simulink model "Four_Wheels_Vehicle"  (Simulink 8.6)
settings: Solver=ode45  StartTime=0.0  StopTime=20  RelTol=1e-3
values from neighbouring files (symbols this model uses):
  beta = 1    [Vehicle_Parameters.m]
  g = 9.81    [Vehicle_Parameters.m]
  H_CoG = 0.700    (= 0.7)    [Vehicle_Parameters.m]
  Hearo = 0.750    (= 0.75)    [Vehicle_Parameters.m]
  Iz = 2480    [Vehicle_Parameters.m]
  Jw = 2.166    [Vehicle_Parameters.m]
  L = 10    [Vehicle_Parameters.m]
  Lf = 1.180    (= 1.18)    [Vehicle_Parameters.m]
  Lr = 1.770    (= 1.77)    [Vehicle_Parameters.m]
  Lw = 1.880    (= 1.88)    [Vehicle_Parameters.m]
  m = 1500    [Vehicle_Parameters.m]
  miu = 0.85    [Vehicle_Parameters.m]
  reff = 0.380    (= 0.38)    [Vehicle_Parameters.m]
undefined symbols (not defined in the file or in its folder): DiscIntNeverNeededParam, Init, Ki, Kp, LowerLimit, sigbuilder_block, Ts, UpperLimit
libraries: simulink x15, powerlib_extras x3
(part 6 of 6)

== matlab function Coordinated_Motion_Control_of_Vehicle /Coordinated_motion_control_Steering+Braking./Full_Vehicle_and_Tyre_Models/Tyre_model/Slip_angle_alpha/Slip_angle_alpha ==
% =================================================================================================================================
% Function: Slip_angle_alpha
% Version:  0.00
% Since:    25 May 2016
% Author:   T.C. Lin
% Input:	x_Vel, y_Vel, yaw_rate, Lf, Lr, deltaw
% Output:	alpha_FL, alpha_FR, alpha_RL, alpha_RR
% Timing:   TBD
% Description: NA
% =================================================================================================================================

function [alpha_FL, alpha_FR, alpha_RL, alpha_RR] = Slip_angle(x_Vel, y_Vel, yaw_rate, Lf, Lr, deltaw)
%# codegen

% % ===== Slip angles at the front tire =====
% 
% % Slip angles at the front left tire
% alpha_FL = deltaw-atan(y_Vel+Lf*yaw_rate/x_Vel);
% 
% % Slip angles at the front right tire
% alpha_FR = deltaw-atan(y_Vel+Lf*yaw_rate/x_Vel);
% 
% 
% % ===== Slip angles at the rear tire =====
% 
% % Slip angles at the rear left tire
% alpha_RL = -atan(y_Vel-Lr*yaw_rate/x_Vel);
% 
% % Slip angles at the rear right tire
% alpha_RR = -atan(y_Vel-Lr*yaw_rate/x_Vel);



alpha_FL=deltaw-atan((y_Vel+Lf*yaw_rate)/(x_Vel-1.65*yaw_rate/2));
alpha_FR=deltaw-atan((y_Vel+Lf*yaw_rate)/(x_Vel+1.65*yaw_rate/2));
alpha_RL=-atan((y_Vel-Lr*yaw_rate)/(x_Vel-1.65*yaw_rate/2));
alpha_RR=-atan((y_Vel-Lr*yaw_rate)/(x_Vel+1.65*yaw_rate/2));

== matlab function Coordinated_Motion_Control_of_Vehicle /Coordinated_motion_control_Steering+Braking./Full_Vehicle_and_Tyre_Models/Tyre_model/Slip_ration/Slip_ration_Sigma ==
% =================================================================================================================================
% Function: Slip_Ration_Sigma
% Version:  0.00
% Since:    24 May 2016
% Author:   T.C. Lin
% Input:	Omega_FL, Omega_FR, Omega_RL, Omega_RR, x_Vel, reff
% Output:	Sigma_FL, Sigma_FR, Sigma_RL, Sigma_RR
% Timing:   TBD
% Description: NA
% =================================================================================================================================

function [Sigma_FL, Sigma_FR, Sigma_RL, Sigma_RR] = Slip_Ration(Omega_FL, Omega_FR, Omega_RL, Omega_RR, x_Vel, reff)
%#codegen

Sigma_FL = (reff*Omega_FL - x_Vel)/(x_Vel);
Sigma_FR = (reff*Omega_FR - x_Vel)/(x_Vel);

Sigma_RL = (reff*Omega_RL - x_Vel)/(x_Vel);
Sigma_RR = (reff*Omega_RR - x_Vel)/(x_Vel);

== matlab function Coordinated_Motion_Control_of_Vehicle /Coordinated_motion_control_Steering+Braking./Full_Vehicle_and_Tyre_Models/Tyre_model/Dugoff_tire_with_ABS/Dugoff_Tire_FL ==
% ================================================================================
% Function: Dugoff_Tire_FL
% Version:  0.00
% Since:    24 May 2016
% Author:   T.C. Lin
% Input:	Sigma, Fz_FL, alpha_FL, miu
% Output:	Fx_FL, Fy_FL
% Timing:   TBD
% Description: NA
% ================================================================================

function [Fx_FL, Fy_FL] = Dugoff_Tire_FL(Sigma, Fz_FL, alpha_FL, miu)
%# codegen

% Cornering stiffness of the tire
Cs = 20000;

% Longitudinal stiffness of the tire
C_alpha = 80000;

% Dugoff's tire model with a variable lamda in the wheel model
Lamda = miu*Fz_FL*(1+Sigma)/(2*sqrt((Cs*Sigma)^2+(C_alpha*(tan(alpha_FL)))^2));

if Lamda < 1
    
    f = Lamda*(2-Lamda);
    
else
    f = 1;
    
end

% Longitudinal tire force
Fx_FL = Cs*Sigma*f/(1+Sigma);

% Lateral tire force
Fy_FL = C_alpha*tan(alpha_FL)*f/(1+Sigma);

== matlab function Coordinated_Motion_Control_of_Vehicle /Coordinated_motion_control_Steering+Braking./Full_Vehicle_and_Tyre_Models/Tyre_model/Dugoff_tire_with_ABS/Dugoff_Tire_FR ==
% ================================================================================
% Function: Dugoff_Tire_FR
% Version:  0.00
% Since:    24 May 2016
% Author:   T.C. Lin
% Input:	Sigma, Fz_FL, alpha_FL, miu
% Output:	Fx_FL, Fy_FL
% Timing:   TBD
% Description: NA
% ================================================================================

function [Fx_FR, Fy_FR] = Dugoff_Tire_FR(Sigma, Fz_FR, alpha_FR, miu)
%# codegen

% Cornering stiffness of the tire
Cs = 20000;

% Longitudinal stiffness of the tire
C_alpha = 80000;

% Dugoff's tire model with a variable lamda in the wheel model
Lamda = miu*Fz_FR*(1+Sigma)/(2*sqrt((Cs*Sigma)^2+(C_alpha*(tan(alpha_FR)))^2));

if Lamda < 1
    
    f = Lamda*(2-Lamda);
    
else   
    f = 1;
    
end

% Longitudinal tire force
Fx_FR = Cs*Sigma*f/(1+Sigma);

% Lateral tire force
Fy_FR = C_alpha*tan(alpha_FR)*f/(1+Sigma);

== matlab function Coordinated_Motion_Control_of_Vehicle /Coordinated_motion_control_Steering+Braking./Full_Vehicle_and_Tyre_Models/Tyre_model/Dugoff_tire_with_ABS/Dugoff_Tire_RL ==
% ================================================================================
% Function: Dugoff_Tire_RL
% Version:  0.00
% Since:    24 May 2016
% Author:   T.C. Lin
% Input:	Sigma, Fz_FL, alpha_FL, miu
% Output:	Fx_FL, Fy_FL
% Timing:   TBD
% Description: NA
% ================================================================================

function [Fx_RL, Fy_RL] = Dugoff_Tire_RL(Sigma, Fz_RL, alpha_RL, miu)
%# codegen

% Cornering stiffness of the tire
Cs = 20000;

% Longitudinal stiffness of the tire
C_alpha = 80000;

% Dugoff's tire model with a variable lamda in the wheel model
Lamda = miu*Fz_RL*(1+Sigma)/(2*sqrt((Cs*Sigma)^2+(C_alpha*(tan(alpha_RL)))^2));

if Lamda < 1
    
    f = Lamda*(2-Lamda);
    
else
    f = 1;
    
end

% Longitudinal tire force
Fx_RL = Cs*Sigma*f/(1+Sigma);

% Lateral tire force
Fy_RL = C_alpha*tan(alpha_RL)*f/(1+Sigma);

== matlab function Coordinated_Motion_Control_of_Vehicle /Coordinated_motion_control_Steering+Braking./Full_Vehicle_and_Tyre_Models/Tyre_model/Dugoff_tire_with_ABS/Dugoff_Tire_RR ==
% ================================================================================
% Function: Dugoff_Tire_RR
% Version:  0.00
% Since:    24 May 2016
% Author:   T.C. Lin
% Input:	Sigma, Fz_FL, alpha_FL, miu
% Output:	Fx_FL, Fy_FL
% Timing:   TBD
% Description: NA
% ================================================================================

function [Fx_RR, Fy_RR] = Dugoff_Tire_RR(Sigma, Fz_RR, alpha_RR, miu)
%# codegen

% Cornering stiffness of the tire
Cs = 20000;

% Longitudinal stiffness of the tire
C_alpha = 80000;

% Dugoff's tire model with a variable lamda in the wheel model
Lamda = miu*Fz_RR*(1+Sigma)/(2*sqrt((Cs*Sigma)^2+(C_alpha*(tan(alpha_RR)))^2));

if Lamda<1
    
    f = Lamda*(2-Lamda);
    
else   
    f = 1;
    
end

% Longitudinal tire force
Fx_RR = Cs*Sigma*f/(1+Sigma);

% Lateral tire force
Fy_RR = C_alpha*tan(alpha_RR)*f/(1+Sigma);

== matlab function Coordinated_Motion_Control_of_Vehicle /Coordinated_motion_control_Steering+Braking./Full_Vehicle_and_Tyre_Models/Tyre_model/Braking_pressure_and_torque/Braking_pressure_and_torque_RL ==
% ================================================================================
% Function: Dugoff_Tire_FL
% Version:  0.00
% Since:    24 May 2016
% Author:   T.C. Lin
% Input:	Sigma, Fz_FL, alpha_FL, miu
% Output:	Fx_FL, Fy_FL
% Timing:   TBD
% Description: NA
% ================================================================================

function [P_RL, Tb_RL] = Dugoff_Tire_RL(M, reff, tw)
%# codegen

% Brake gain
Kb = 1;

% Dugoff's tire model with a variable lamda in the wheel model
P_RL = -2*M*reff/(Kb*tw);

Tb_RL=Kb*P_RL;

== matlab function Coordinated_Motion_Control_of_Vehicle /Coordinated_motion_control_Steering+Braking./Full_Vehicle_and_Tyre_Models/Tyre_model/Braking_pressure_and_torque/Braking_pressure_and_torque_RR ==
% ================================================================================
% Function: Dugoff_Tire_FL
% Version:  0.00
% Since:    24 May 2016
% Author:   T.C. Lin
% Input:	Sigma, Fz_FL, alpha_FL, miu
% Output:	Fx_FL, Fy_FL
% Timing:   TBD
% Description: NA
% ================================================================================

function [P_RR, Tb_RR] = Dugoff_Tire_FL(M, reff, tw)
%# codegen

% Brake gain
Kb = 1;

% Dugoff's tire model with a variable lamda in the wheel model
P_RR = 2*M*reff/(Kb*tw);

Tb_RR=Kb*P_RR;

== matlab function Coordinated_Motion_Control_of_Vehicle /Coordinated_motion_control_Steering+Braking./Motion_Coordinator/Controller_and_actuator
Steering_and_Braking/Brake_controller_1/Brake_Actuator_1/Actuator/LPF ==
function out = lpf(in1,in2,f)

    temp=1e4/2/pi/f;
    out=(in2*temp+in1)/(temp+1);

== matlab function Coordinated_Motion_Control_of_Vehicle /Coordinated_motion_control_Steering+Braking./Motion_Coordinator/Controller_and_actuator
Steering_and_Braking/Steering_controller/Steering_Actuator/Actuator/LPF ==
function out = lpf(in1,in2,f)

    temp=1e4/2/pi/f;
    out=(in2*temp+in1)/(temp+1);

== matlab function Coordinated_Motion_Control_of_Vehicle /Coordinated_motion_control_Steering+Braking./Motion_Coordinator/Controller_and_actuator
Steering_and_Braking/Brake_controller_2/Brake_Actuator_2/Actuator/LPF ==
function out = lpf(in1,in2,f)

    temp=1e4/2/pi/f;
    out=(in2*temp+in1)/(temp+1);

== matlab function Coordinated_Motion_Control_of_Vehicle /Coordinated_motion_control_Steering+Braking./Motion_Coordinator/Controller_and_actuator
Steering_and_Braking/Brake_controller_3/Brake_Actuator_3/Actuator/LPF ==
function out = lpf(in1,in2,f)

    temp=1e4/2/pi/f;
    out=(in2*temp+in1)/(temp+1);

== matlab function Coordinated_Motion_Control_of_Vehicle /Coordinated_motion_control_Steering+Braking./Motion_Coordinator/Controller_and_actuator
Steering_and_Braking/Brake_controller_4/Brake_Actuator_4/Actuator/LPF ==
function out = lpf(in1,in2,f)

    temp=1e4/2/pi/f;
    out=(in2*temp+in1)/(temp+1);

== matlab function Coordinated_Motion_Control_of_Vehicle /Control_of_braking_without_steering_control./Motion_Coordinator_1/Controller_and_actuator
Steering_and_Braking_1/Brake_controller_1/Brake_Actuator_1/Actuator/LPF ==
function out = lpf(in1,in2,f)

    temp=1e4/2/pi/f;
    out=(in2*temp+in1)/(temp+1);

== matlab function Coordinated_Motion_Control_of_Vehicle /Control_of_braking_without_steering_control./Motion_Coordinator_1/Controller_and_actuator
Steering_and_Braking_1/Brake_controller_2/Brake_Actuator_2/Actuator/LPF ==
function out = lpf(in1,in2,f)

    temp=1e4/2/pi/f;
    out=(in2*temp+in1)/(temp+1);

== matlab function Coordinated_Motion_Control_of_Vehicle /Control_of_braking_without_steering_control./Motion_Coordinator_1/Controller_and_actuator
Steering_and_Braking_1/Brake_controller_3/Brake_Actuator_3/Actuator/LPF ==
function out = lpf(in1,in2,f)

    temp=1e4/2/pi/f;
    out=(in2*temp+in1)/(temp+1);

== matlab function Coordinated_Motion_Control_of_Vehicle /Control_of_braking_without_steering_control./Motion_Coordinator_1/Controller_and_actuator
Steering_and_Braking_1/Brake_controller_4/Brake_Actuator_4/Actuator/LPF ==
function out = lpf(in1,in2,f)

    temp=1e4/2/pi/f;
    out=(in2*temp+in1)/(temp+1);

== matlab function Coordinated_Motion_Control_of_Vehicle /Control_of_braking_without_steering_control./Motion_Coordinator_1/Controller_and_actuator
Steering_and_Braking_1/Steering_controller/Steering_Actuator/Actuator/LPF ==
function out = lpf(in1,in2,f)

    temp=1e4/2/pi/f;
    out=(in2*temp+in1)/(temp+1);

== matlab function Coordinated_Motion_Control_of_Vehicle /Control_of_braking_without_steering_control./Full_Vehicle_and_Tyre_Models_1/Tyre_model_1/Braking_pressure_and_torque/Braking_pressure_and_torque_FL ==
% ================================================================================
% Function: Dugoff_Tire_FL
% Version:  0.00
% Since:    24 May 2016
% Author:   T.C. Lin
% Input:	Sigma, Fz_FL, alpha_FL, miu
% Output:	Fx_FL, Fy_FL
% Timing:   TBD
% Description: NA
% ================================================================================

function [P_FL, Tb_FL]  = Dugoff_Tire_FL(M, reff, tw, SteeringAng)
%# codegen

% Brake gain
Kb = 100;

% Dugoff's tire model with a variable lamda in the wheel model
P_FL = -2*M*reff/(Kb*tw)*cos(SteeringAng);

Tb_FL=Kb*P_FL;

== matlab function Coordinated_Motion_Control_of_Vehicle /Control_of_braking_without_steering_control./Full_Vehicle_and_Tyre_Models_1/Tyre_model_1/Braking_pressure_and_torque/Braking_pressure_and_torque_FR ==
% ================================================================================
% Function: Dugoff_Tire_FL
% Version:  0.00
% Since:    24 May 2016
% Author:   T.C. Lin
% Input:	Sigma, Fz_FL, alpha_FL, miu
% Output:	Fx_FL, Fy_FL
% Timing:   TBD
% Description: NA
% ================================================================================

function [P_FR, Tb_FR] = Dugoff_Tire_FL(M, reff, tw, SteeringAng)
%# codegen

% Brake gain
Kb = 100;

% Dugoff's tire model with a variable lamda in the wheel model
P_FR = 2*M*reff/(Kb*tw)*cos(SteeringAng);

Tb_FR=Kb*P_FR;

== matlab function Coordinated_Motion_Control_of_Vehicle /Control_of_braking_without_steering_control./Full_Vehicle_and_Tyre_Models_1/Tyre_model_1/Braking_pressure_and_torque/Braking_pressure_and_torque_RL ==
% ================================================================================
% Function: Dugoff_Tire_FL
% Version:  0.00
% Since:    24 May 2016
% Author:   T.C. Lin
% Input:	Sigma, Fz_FL, alpha_FL, miu
% Output:	Fx_FL, Fy_FL
% Timing:   TBD
% Description: NA
% ================================================================================

function [P_RL, Tb_RL] = Dugoff_Tire_RL(M, reff, tw)
%# codegen

% Brake gain
Kb = 1;

% Dugoff's tire model with a variable lamda in the wheel model
P_RL = -2*M*reff/(Kb*tw);

Tb_RL=Kb*P_RL;

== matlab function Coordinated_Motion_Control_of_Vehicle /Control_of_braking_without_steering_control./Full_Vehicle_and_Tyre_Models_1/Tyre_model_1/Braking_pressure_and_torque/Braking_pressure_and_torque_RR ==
% ================================================================================
% Function: Dugoff_Tire_FL
% Version:  0.00
% Since:    24 May 2016
% Author:   T.C. Lin
% Input:	Sigma, Fz_FL, alpha_FL, miu
% Output:	Fx_FL, Fy_FL
% Timing:   TBD
% Description: NA
% ================================================================================

function [P_RR, Tb_RR] = Dugoff_Tire_FL(M, reff, tw)
%# codegen

% Brake gain
Kb = 1;

% Dugoff's tire model with a variable lamda in the wheel model
P_RR = 2*M*reff/(Kb*tw);

Tb_RR=Kb*P_RR;

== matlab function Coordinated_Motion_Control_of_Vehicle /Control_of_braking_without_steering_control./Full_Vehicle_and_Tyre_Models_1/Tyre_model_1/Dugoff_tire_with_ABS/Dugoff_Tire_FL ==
% ================================================================================
% Function: Dugoff_Tire_FL
% Version:  0.00
% Since:    24 May 2016
% Author:   T.C. Lin
% Input:	Sigma, Fz_FL, alpha_FL, miu
% Output:	Fx_FL, Fy_FL
% Timing:   TBD
% Description: NA
% ================================================================================

function [Fx_FL, Fy_FL] = Dugoff_Tire_FL(Sigma, Fz_FL, alpha_FL, miu)
%# codegen

% Cornering stiffness of the tire
Cs = 20000;

% Longitudinal stiffness of the tire
C_alpha = 80000;

% Dugoff's tire model with a variable lamda in the wheel model
Lamda = miu*Fz_FL*(1+Sigma)/(2*sqrt((Cs*Sigma)^2+(C_alpha*(tan(alpha_FL)))^2));

if Lamda < 1
    
    f = Lamda*(2-Lamda);
    
else
    f = 1;
    
end

% Longitudinal tire force
Fx_FL = Cs*Sigma*f/(1+Sigma);

% Lateral tire force
Fy_FL = C_alpha*tan(alpha_FL)*f/(1+Sigma);

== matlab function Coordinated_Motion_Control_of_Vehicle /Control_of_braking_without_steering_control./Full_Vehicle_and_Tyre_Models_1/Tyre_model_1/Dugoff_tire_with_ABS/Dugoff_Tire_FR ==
% ================================================================================
% Function: Dugoff_Tire_FR
% Version:  0.00
% Since:    24 May 2016
% Author:   T.C. Lin
% Input:	Sigma, Fz_FL, alpha_FL, miu
% Output:	Fx_FL, Fy_FL
% Timing:   TBD
% Description: NA
% ================================================================================

function [Fx_FR, Fy_FR] = Dugoff_Tire_FR(Sigma, Fz_FR, alpha_FR, miu)
%# codegen

% Cornering stiffness of the tire
Cs = 20000;

% Longitudinal stiffness of the tire
C_alpha = 80000;

% Dugoff's tire model with a variable lamda in the wheel model
Lamda = miu*Fz_FR*(1+Sigma)/(2*sqrt((Cs*Sigma)^2+(C_alpha*(tan(alpha_FR)))^2));

if Lamda < 1
    
    f = Lamda*(2-Lamda);
    
else   
    f = 1;
    
end

% Longitudinal tire force
Fx_FR = Cs*Sigma*f/(1+Sigma);

% Lateral tire force
Fy_FR = C_alpha*tan(alpha_FR)*f/(1+Sigma);

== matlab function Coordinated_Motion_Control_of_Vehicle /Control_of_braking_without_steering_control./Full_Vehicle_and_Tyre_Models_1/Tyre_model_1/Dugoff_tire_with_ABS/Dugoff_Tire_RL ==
% ================================================================================
% Function: Dugoff_Tire_RL
% Version:  0.00
% Since:    24 May 2016
% Author:   T.C. Lin
% Input:	Sigma, Fz_FL, alpha_FL, miu
% Output:	Fx_FL, Fy_FL
% Timing:   TBD
% Description: NA
% ================================================================================

function [Fx_RL, Fy_RL] = Dugoff_Tire_RL(Sigma, Fz_RL, alpha_RL, miu)
%# codegen

% Cornering stiffness of the tire
Cs = 20000;

% Longitudinal stiffness of the tire
C_alpha = 80000;

% Dugoff's tire model with a variable lamda in the wheel model
Lamda = miu*Fz_RL*(1+Sigma)/(2*sqrt((Cs*Sigma)^2+(C_alpha*(tan(alpha_RL)))^2));

if Lamda < 1
    
    f = Lamda*(2-Lamda);
    
else
    f = 1;
    
end

% Longitudinal tire force
Fx_RL = Cs*Sigma*f/(1+Sigma);

% Lateral tire force
Fy_RL = C_alpha*tan(alpha_RL)*f/(1+Sigma);

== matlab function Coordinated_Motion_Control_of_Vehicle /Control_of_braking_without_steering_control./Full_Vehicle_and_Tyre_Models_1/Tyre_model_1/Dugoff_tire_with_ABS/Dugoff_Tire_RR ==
% ================================================================================
% Function: Dugoff_Tire_RR
% Version:  0.00
% Since:    24 May 2016
% Author:   T.C. Lin
% Input:	Sigma, Fz_FL, alpha_FL, miu
% Output:	Fx_FL, Fy_FL
% Timing:   TBD
% Description: NA
% ================================================================================

function [Fx_RR, Fy_RR] = Dugoff_Tire_RR(Sigma, Fz_RR, alpha_RR, miu)
%# codegen

% Cornering stiffness of the tire
Cs = 20000;

% Longitudinal stiffness of the tire
C_alpha = 80000;

% Dugoff's tire model with a variable lamda in the wheel model
Lamda = miu*Fz_RR*(1+Sigma)/(2*sqrt((Cs*Sigma)^2+(C_alpha*(tan(alpha_RR)))^2));

if Lamda<1
    
    f = Lamda*(2-Lamda);
    
else   
    f = 1;
    
end

% Longitudinal tire force
Fx_RR = Cs*Sigma*f/(1+Sigma);

% Lateral tire force
Fy_RR = C_alpha*tan(alpha_RR)*f/(1+Sigma);

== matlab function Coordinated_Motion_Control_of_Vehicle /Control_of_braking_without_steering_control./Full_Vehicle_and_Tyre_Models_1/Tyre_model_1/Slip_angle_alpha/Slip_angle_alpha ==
% =================================================================================================================================
% Function: Slip_angle_alpha
% Version:  0.00
% Since:    25 May 2016
% Author:   T.C. Lin
% Input:	x_Vel, y_Vel, yaw_rate, Lf, Lr, deltaw
% Output:	alpha_FL, alpha_FR, alpha_RL, alpha_RR
% Timing:   TBD
% Description: NA
% =================================================================================================================================

function [alpha_FL, alpha_FR, alpha_RL, alpha_RR] = Slip_angle(x_Vel, y_Vel, yaw_rate, Lf, Lr, deltaw)
%# codegen

% % ===== Slip angles at the front tire =====

% % Slip angles at the front left tire
% alpha_FL = deltaw-atan(y_Vel+Lf*yaw_rate/x_Vel);
% 
% % Slip angles at the front right tire
% alpha_FR = deltaw-atan(y_Vel+Lf*yaw_rate/x_Vel);
% 
% 
% % ===== Slip angles at the rear tire =====
% 
% % Slip angles at the rear left tire
% alpha_RL = -atan(y_Vel-Lr*yaw_rate/x_Vel);
% 
% % Slip angles at the rear right tire
% alpha_RR = -atan(y_Vel-Lr*yaw_rate/x_Vel);



alpha_FL=deltaw-atan((y_Vel+Lf*yaw_rate)/(x_Vel-1.65*yaw_rate/2));
alpha_FR=deltaw-atan((y_Vel+Lf*yaw_rate)/(x_Vel+1.65*yaw_rate/2));
alpha_RL=-atan((y_Vel-Lr*yaw_rate)/(x_Vel-1.65*yaw_rate/2));
alpha_RR=-atan((y_Vel-Lr*yaw_rate)/(x_Vel+1.65*yaw_rate/2));

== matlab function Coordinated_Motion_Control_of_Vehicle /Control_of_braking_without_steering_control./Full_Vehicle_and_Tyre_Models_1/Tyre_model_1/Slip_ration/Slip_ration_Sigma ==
% =================================================================================================================================
% Function: Slip_Ration_Sigma
% Version:  0.00
% Since:    24 May 2016
% Author:   T.C. Lin
% Input:	Omega_FL, Omega_FR, Omega_RL, Omega_RR, x_Vel, reff
% Output:	Sigma_FL, Sigma_FR, Sigma_RL, Sigma_RR
% Timing:   TBD
% Description: NA
% =================================================================================================================================

function [Sigma_FL, Sigma_FR, Sigma_RL, Sigma_RR] = Slip_Ration(Omega_FL, Omega_FR, Omega_RL, Omega_RR, x_Vel, reff)
%#codegen

Sigma_FL = (reff*Omega_FL - x_Vel)/(x_Vel);
Sigma_FR = (reff*Omega_FR - x_Vel)/(x_Vel);

Sigma_RL = (reff*Omega_RL - x_Vel)/(x_Vel);
Sigma_RR = (reff*Omega_RR - x_Vel)/(x_Vel);

== matlab function Coordinated_Motion_Control_of_Vehicle /Control_of_steering_without_braking_control./Motion_Coordinator_2/Controller_and_actuator
Steering_and_Braking_2/Brake_controller_1/Brake_Actuator_1/Actuator/LPF ==
function out = lpf(in1,in2,f)

    temp=1e4/2/pi/f;
    out=(in2*temp+in1)/(temp+1);

== matlab function Coordinated_Motion_Control_of_Vehicle /Control_of_steering_without_braking_control./Motion_Coordinator_2/Controller_and_actuator
Steering_and_Braking_2/Brake_controller_2/Brake_Actuator_2/Actuator/LPF ==
function out = lpf(in1,in2,f)

    temp=1e4/2/pi/f;
    out=(in2*temp+in1)/(temp+1);

== matlab function Coordinated_Motion_Control_of_Vehicle /Control_of_steering_without_braking_control./Motion_Coordinator_2/Controller_and_actuator
Steering_and_Braking_2/Brake_controller_3/Brake_Actuator_3/Actuator/LPF ==
function out = lpf(in1,in2,f)

    temp=1e4/2/pi/f;
    out=(in2*temp+in1)/(temp+1);

== matlab function Coordinated_Motion_Control_of_Vehicle /Control_of_steering_without_braking_control./Motion_Coordinator_2/Controller_and_actuator
Steering_and_Braking_2/Brake_controller_4/Brake_Actuator_4/Actuator/LPF ==
function out = lpf(in1,in2,f)

    temp=1e4/2/pi/f;
    out=(in2*temp+in1)/(temp+1);

== matlab function Coordinated_Motion_Control_of_Vehicle /Control_of_steering_without_braking_control./Motion_Coordinator_2/Controller_and_actuator
Steering_and_Braking_2/Steering_controller/Steering_Actuator/Actuator/LPF ==
function out = lpf(in1,in2,f)

    temp=1e4/2/pi/f;
    out=(in2*temp+in1)/(temp+1);

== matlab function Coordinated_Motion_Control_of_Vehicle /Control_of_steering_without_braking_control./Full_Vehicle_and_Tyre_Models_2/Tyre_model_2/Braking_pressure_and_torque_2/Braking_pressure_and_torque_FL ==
% ================================================================================
% Function: Dugoff_Tire_FL
% Version:  0.00
% Since:    24 May 2016
% Author:   T.C. Lin
% Input:	Sigma, Fz_FL, alpha_FL, miu
% Output:	Fx_FL, Fy_FL
% Timing:   TBD
% Description: NA
% ================================================================================

function [P_FL, Tb_FL]  = Dugoff_Tire_FL(M, reff, tw, SteeringAng)
%# codegen

% Brake gain
Kb = 100;

% Dugoff's tire model with a variable lamda in the wheel model
P_FL = -2*M*reff/(Kb*tw)*cos(SteeringAng);

Tb_FL=Kb*P_FL;

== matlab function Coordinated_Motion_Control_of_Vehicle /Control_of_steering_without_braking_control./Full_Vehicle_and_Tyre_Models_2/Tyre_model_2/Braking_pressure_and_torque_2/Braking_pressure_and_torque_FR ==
% ================================================================================
% Function: Dugoff_Tire_FL
% Version:  0.00
% Since:    24 May 2016
% Author:   T.C. Lin
% Input:	Sigma, Fz_FL, alpha_FL, miu
% Output:	Fx_FL, Fy_FL
% Timing:   TBD
% Description: NA
% ================================================================================

function [P_FR, Tb_FR] = Dugoff_Tire_FL(M, reff, tw, SteeringAng)
%# codegen

% Brake gain
Kb = 100;

% Dugoff's tire model with a variable lamda in the wheel model
P_FR = 2*M*reff/(Kb*tw)*cos(SteeringAng);

Tb_FR=Kb*P_FR;

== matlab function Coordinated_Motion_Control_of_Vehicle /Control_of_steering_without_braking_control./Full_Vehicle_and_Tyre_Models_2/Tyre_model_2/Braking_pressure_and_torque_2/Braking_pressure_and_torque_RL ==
% ================================================================================
% Function: Dugoff_Tire_FL
% Version:  0.00
% Since:    24 May 2016
% Author:   T.C. Lin
% Input:	Sigma, Fz_FL, alpha_FL, miu
% Output:	Fx_FL, Fy_FL
% Timing:   TBD
% Description: NA
% ================================================================================

function [P_RL, Tb_RL] = Dugoff_Tire_RL(M, reff, tw)
%# codegen

% Brake gain
Kb = 1;

% Dugoff's tire model with a variable lamda in the wheel model
P_RL = -2*M*reff/(Kb*tw);

Tb_RL=Kb*P_RL;

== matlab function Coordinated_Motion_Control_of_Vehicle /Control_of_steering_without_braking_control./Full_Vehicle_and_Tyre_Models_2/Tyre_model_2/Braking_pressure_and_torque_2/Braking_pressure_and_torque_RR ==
% ================================================================================
% Function: Dugoff_Tire_FL
% Version:  0.00
% Since:    24 May 2016
% Author:   T.C. Lin
% Input:	Sigma, Fz_FL, alpha_FL, miu
% Output:	Fx_FL, Fy_FL
% Timing:   TBD
% Description: NA
% ================================================================================

function [P_RR, Tb_RR] = Dugoff_Tire_FL(M, reff, tw)
%# codegen

% Brake gain
Kb = 1;

% Dugoff's tire model with a variable lamda in the wheel model
P_RR = 2*M*reff/(Kb*tw);

Tb_RR=Kb*P_RR;

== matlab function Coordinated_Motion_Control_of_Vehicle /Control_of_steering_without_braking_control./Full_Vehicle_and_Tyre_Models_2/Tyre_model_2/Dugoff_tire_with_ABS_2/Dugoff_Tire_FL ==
% ================================================================================
% Function: Dugoff_Tire_FL
% Version:  0.00
% Since:    24 May 2016
% Author:   T.C. Lin
% Input:	Sigma, Fz_FL, alpha_FL, miu
% Output:	Fx_FL, Fy_FL
% Timing:   TBD
% Description: NA
% ================================================================================

function [Fx_FL, Fy_FL] = Dugoff_Tire_FL(Sigma, Fz_FL, alpha_FL, miu)
%# codegen

% Cornering stiffness of the tire
Cs = 20000;

% Longitudinal stiffness of the tire
C_alpha = 80000;

% Dugoff's tire model with a variable lamda in the wheel model
Lamda = miu*Fz_FL*(1+Sigma)/(2*sqrt((Cs*Sigma)^2+(C_alpha*(tan(alpha_FL)))^2));

if Lamda < 1
    
    f = Lamda*(2-Lamda);
    
else
    f = 1;
    
end

% Longitudinal tire force
Fx_FL = Cs*Sigma*f/(1+Sigma);

% Lateral tire force
Fy_FL = C_alpha*tan(alpha_FL)*f/(1+Sigma);

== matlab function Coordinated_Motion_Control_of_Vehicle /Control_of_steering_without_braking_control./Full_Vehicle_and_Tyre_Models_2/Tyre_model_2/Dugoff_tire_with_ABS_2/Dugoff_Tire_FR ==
% ================================================================================
% Function: Dugoff_Tire_FR
% Version:  0.00
% Since:    24 May 2016
% Author:   T.C. Lin
% Input:	Sigma, Fz_FL, alpha_FL, miu
% Output:	Fx_FL, Fy_FL
% Timing:   TBD
% Description: NA
% ================================================================================

function [Fx_FR, Fy_FR] = Dugoff_Tire_FR(Sigma, Fz_FR, alpha_FR, miu)
%# codegen

% Cornering stiffness of the tire
Cs = 20000;

% Longitudinal stiffness of the tire
C_alpha = 80000;

% Dugoff's tire model with a variable lamda in the wheel model
Lamda = miu*Fz_FR*(1+Sigma)/(2*sqrt((Cs*Sigma)^2+(C_alpha*(tan(alpha_FR)))^2));

if Lamda < 1
    
    f = Lamda*(2-Lamda);
    
else   
    f = 1;
    
end

% Longitudinal tire force
Fx_FR = Cs*Sigma*f/(1+Sigma);

% Lateral tire force
Fy_FR = C_alpha*tan(alpha_FR)*f/(1+Sigma);

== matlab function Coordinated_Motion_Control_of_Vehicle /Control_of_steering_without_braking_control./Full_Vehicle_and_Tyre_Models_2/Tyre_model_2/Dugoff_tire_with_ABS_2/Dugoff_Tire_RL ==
% ================================================================================
% Function: Dugoff_Tire_RL
% Version:  0.00
% Since:    24 May 2016
% Author:   T.C. Lin
% Input:	Sigma, Fz_FL, alpha_FL, miu
% Output:	Fx_FL, Fy_FL
% Timing:   TBD
% Description: NA
% ================================================================================

function [Fx_RL, Fy_RL] = Dugoff_Tire_RL(Sigma, Fz_RL, alpha_RL, miu)
%# codegen

% Cornering stiffness of the tire
Cs = 20000;

% Longitudinal stiffness of the tire
C_alpha = 80000;

% Dugoff's tire model with a variable lamda in the wheel model
Lamda = miu*Fz_RL*(1+Sigma)/(2*sqrt((Cs*Sigma)^2+(C_alpha*(tan(alpha_RL)))^2));

if Lamda < 1
    
    f = Lamda*(2-Lamda);
    
else
    f = 1;
    
end

% Longitudinal tire force
Fx_RL = Cs*Sigma*f/(1+Sigma);

% Lateral tire force
Fy_RL = C_alpha*tan(alpha_RL)*f/(1+Sigma);

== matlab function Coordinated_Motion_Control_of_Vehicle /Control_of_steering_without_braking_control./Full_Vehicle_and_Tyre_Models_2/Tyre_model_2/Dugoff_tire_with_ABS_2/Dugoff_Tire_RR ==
% ================================================================================
% Function: Dugoff_Tire_RR
% Version:  0.00
% Since:    24 May 2016
% Author:   T.C. Lin
% Input:	Sigma, Fz_FL, alpha_FL, miu
% Output:	Fx_FL, Fy_FL
% Timing:   TBD
% Description: NA
% ================================================================================

function [Fx_RR, Fy_RR] = Dugoff_Tire_RR(Sigma, Fz_RR, alpha_RR, miu)
%# codegen

% Cornering stiffness of the tire
Cs = 20000;

% Longitudinal stiffness of the tire
C_alpha = 80000;

% Dugoff's tire model with a variable lamda in the wheel model
Lamda = miu*Fz_RR*(1+Sigma)/(2*sqrt((Cs*Sigma)^2+(C_alpha*(tan(alpha_RR)))^2));

if Lamda<1
    
    f = Lamda*(2-Lamda);
    
else   
    f = 1;
    
end

% Longitudinal tire force
Fx_RR = Cs*Sigma*f/(1+Sigma);

% Lateral tire force
Fy_RR = C_alpha*tan(alpha_RR)*f/(1+Sigma);

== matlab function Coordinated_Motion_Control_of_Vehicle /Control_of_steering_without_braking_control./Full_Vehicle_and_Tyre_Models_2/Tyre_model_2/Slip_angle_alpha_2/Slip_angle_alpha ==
% =================================================================================================================================
% Function: Slip_angle_alpha
% Version:  0.00
% Since:    25 May 2016
% Author:   T.C. Lin
% Input:	x_Vel, y_Vel, yaw_rate, Lf, Lr, deltaw
% Output:	alpha_FL, alpha_FR, alpha_RL, alpha_RR
% Timing:   TBD
% Description: NA
% =================================================================================================================================

function [alpha_FL, alpha_FR, alpha_RL, alpha_RR] = Slip_angle(x_Vel, y_Vel, yaw_rate, Lf, Lr, deltaw)
%# codegen

% % ===== Slip angles at the front tire =====

% % Slip angles at the front left tire
% alpha_FL = deltaw-atan(y_Vel+Lf*yaw_rate/x_Vel);
% 
% % Slip angles at the front right tire
% alpha_FR = deltaw-atan(y_Vel+Lf*yaw_rate/x_Vel);
% 
% 
% % ===== Slip angles at the rear tire =====
% 
% % Slip angles at the rear left tire
% alpha_RL = -atan(y_Vel-Lr*yaw_rate/x_Vel);
% 
% % Slip angles at the rear right tire
% alpha_RR = -atan(y_Vel-Lr*yaw_rate/x_Vel);



alpha_FL=deltaw-atan((y_Vel+Lf*yaw_rate)/(x_Vel-1.65*yaw_rate/2));
alpha_FR=deltaw-atan((y_Vel+Lf*yaw_rate)/(x_Vel+1.65*yaw_rate/2));
alpha_RL=-atan((y_Vel-Lr*yaw_rate)/(x_Vel-1.65*yaw_rate/2));
alpha_RR=-atan((y_Vel-Lr*yaw_rate)/(x_Vel+1.65*yaw_rate/2));

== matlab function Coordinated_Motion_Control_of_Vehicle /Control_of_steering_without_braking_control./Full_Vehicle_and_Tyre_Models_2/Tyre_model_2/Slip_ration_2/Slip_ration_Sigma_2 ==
% =================================================================================================================================
% Function: Slip_Ration_Sigma
% Version:  0.00
% Since:    24 May 2016
% Author:   T.C. Lin
% Input:	Omega_FL, Omega_FR, Omega_RL, Omega_RR, x_Vel, reff
% Output:	Sigma_FL, Sigma_FR, Sigma_RL, Sigma_RR
% Timing:   TBD
% Description: NA
% =================================================================================================================================

function [Sigma_FL, Sigma_FR, Sigma_RL, Sigma_RR] = Slip_Ration(Omega_FL, Omega_FR, Omega_RL, Omega_RR, x_Vel, reff)
%#codegen

Sigma_FL = (reff*Omega_FL - x_Vel)/(x_Vel);
Sigma_FR = (reff*Omega_FR - x_Vel)/(x_Vel);

Sigma_RL = (reff*Omega_RL - x_Vel)/(x_Vel);
Sigma_RR = (reff*Omega_RR - x_Vel)/(x_Vel);
